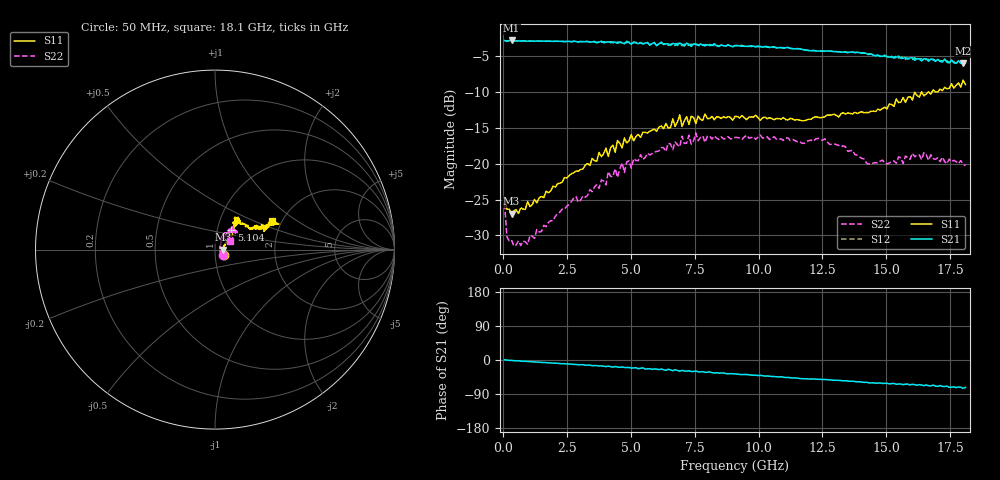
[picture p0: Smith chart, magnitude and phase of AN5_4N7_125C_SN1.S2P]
! Network Analyzer HP8720D.06.14 Serial No. US36140669
!  5 Jul 2005  07:16:07
! Frequency  S11  S21  S12  S22
# HZ  S  DB R 50
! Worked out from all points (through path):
!   201 points, 50 MHz to 18.1 GHz, reference 50 ohm
!   highest |S21| = -2.78 dB at 320.8 MHz (marker M1); lowest = -6.0 dB at 18.01 GHz (marker M2)
!   group delay of S21, straight-line fit = 11.3 ps
!   lowest |S11| = -26.9 dB at 320.8 MHz (marker M3), VSWR 1.09, Z = 54.7 - j0.0475 ohm
!   |S11| at or under -10 dB: start of sweep to 16.11 GHz; 16.11 GHz to 16.38 GHz (264.1 MHz wide, 1.63 % of centre); 16.39 GHz to 16.64 GHz (248.3 MHz wide, 1.5 % of centre)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
!   |S22| runs from -31.5 to -15.7 dB; largest |S21 - S12| = 0.034
!   S11 on the Smith chart (normalised r, x): 50 MHz: 1.11, -0.06; 5.104 GHz: 1.17, +0.27; 18.1 GHz: 1.79, +0.65
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5e7  -24.65 -29.1  -2.80 0.6  -2.82 0.8  -25.57 -37.4
1.4025e8  -26.33 -15.0  -2.91 -0.2  -2.88 -0.2  -30.21 -23.3
3.2075e8  -26.94 -0.6  -2.78 -0.9  -2.83 -0.8  -30.60 -5.3
9.525e8  -25.27 15.9  -2.89 -4.0  -2.84 -3.9  -31.26 22.3
3.1185e9  -20.74 39.4  -2.95 -12.3  -2.99 -12.6  -24.47 54.8
4.021e9  -17.82 44.9  -3.04 -17.3  -3.02 -16.2  -22.93 55.1
4.11125e9  -18.98 45.4  -2.96 -16.1  -3.07 -17.1  -21.09 55.5
4.47225e9  -16.75 43.0  -3.19 -18.3  -2.98 -17.8  -21.90 60.6
4.65275e9  -17.79 43.7  -3.12 -18.4  -3.04 -19.7  -19.88 60.5
4.743e9  -16.39 47.1  -3.23 -19.6  -3.11 -18.8  -21.22 57.0
5.104e9  -16.80 50.7  -2.99 -20.9  -3.11 -21.3  -19.27 53.8
6.09675e9  -14.86 50.4  -3.26 -25.4  -3.15 -25.0  -18.20 52.9
6.909e9  -13.18 53.7  -3.13 -29.5  -3.19 -27.6  -17.64 48.9
6.99925e9  -14.77 54.0  -3.33 -27.6  -3.53 -29.3  -16.12 49.7
7.36025e9  -13.37 49.2  -3.61 -30.3  -3.28 -29.7  -17.26 52.9
7.54075e9  -14.38 51.7  -3.33 -28.9  -3.27 -31.7  -15.71 51.3
9.075e9  -13.37 54.1  -3.51 -36.8  -3.49 -36.8  -16.31 40.9
1.21435e10  -13.56 43.5  -4.20 -50.1  -4.16 -50.2  -16.86 51.0
1.512175e10  -11.64 27.9  -5.12 -63.0  -4.95 -62.4  -19.90 44.1
1.64755e10  -10.53 25.3  -5.34 -67.7  -5.67 -65.9  -18.43 28.4
1.800975e10  -8.32 21.7  -5.99 -74.9  -5.88 -74.3  -20.07 36.1
1.81e10  -8.94 26.4  -5.94 -72.5  -6.18 -73.4  -20.25 31.4
